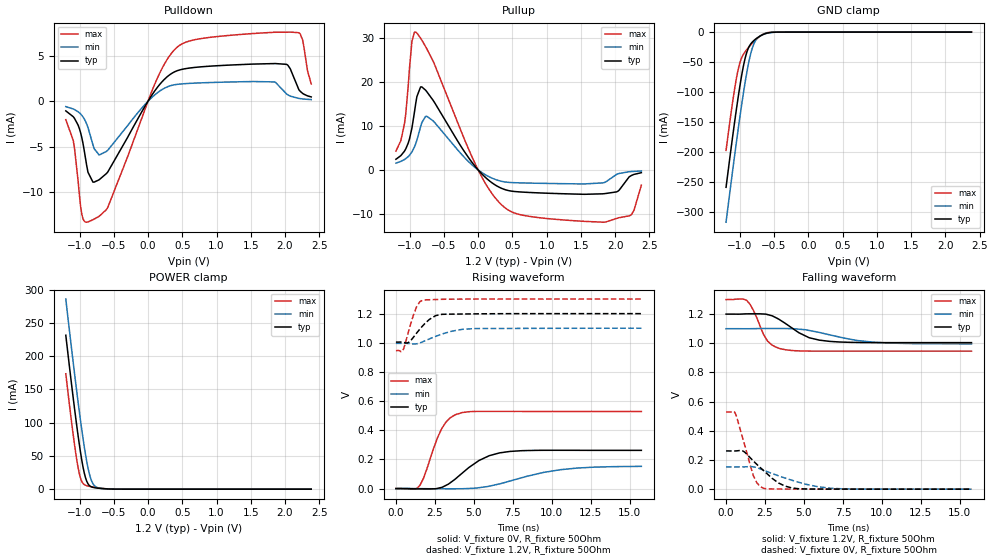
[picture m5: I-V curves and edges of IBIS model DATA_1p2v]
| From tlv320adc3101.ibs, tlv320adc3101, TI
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|   DATA_1p2v
[Model]   DATA_1p2v
Model_type   3-state
Polarity   Non-Inverting
Vmeas = 0.6
Vref = 0
Cref = 5pF
Rref = 1000000
|   typ   min   max
C_comp   1.339pF   1.297pF   1.403pF
[Voltage Range]   1.2   1.1   1.3
[Temperature Range]   27   85   -40
[Pullup Reference]   1.2   1.1   1.3
[Pulldown Reference]   -0   -0   -0
[Power Clamp Reference]   1.2   1.1   1.3
[GND Clamp Reference]   -0   -0   -0
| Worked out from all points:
|   slope of the pulldown table from 0 to 0.18 V, typ, clamps not added: 93.3 ohm
|   slope of the pullup table from 0 to 0.18 V, typ, clamps not added: 67.6 ohm
|   GND clamp passes 1 mA (typ) near -0.57 V on its own axis
|   POWER clamp passes 1 mA (typ) near -0.68 V on its own axis
|   falling waveform, V_fixture 1.2V, R_fixture 50Ohm: 20-80 % time 1.78ns typ, 2.86ns min, 916ps max; typ from 1.2 V to 1 V
|   rising waveform, V_fixture 0V, R_fixture 50Ohm: 20-80 % time 2.02ns typ, 3.54ns min, 1.12ns max; typ from 0 V to 0.262 V
|   rising waveform, V_fixture 1.2V, R_fixture 50Ohm: 20-80 % time 992ps typ, 1.64ns min, 608ps max; typ from 1 V to 1.2 V
|   falling waveform, V_fixture 0V, R_fixture 50Ohm: 20-80 % time 1.63ns typ, 2.66ns min, 845ps max; typ from 0.262 V to 0 V
[Pulldown]
|   Voltage   I(typ)   I(min)   I(max)
-1.2V     -1.067mA   -596.5uA   -2.034mA
-1.092V   -1.704mA   -854.7uA   -4.302mA
-1.02V    -2.641mA   -1.168mA   -8.814mA
-966mV    -4.025mA   -1.562mA   -12.47mA
-894mV    -7.132mA   -2.535mA   -13.33mA
-714mV    -8.661mA   -5.927mA   -12.69mA
-588mV    -7.809mA   -5.412mA   -11.72mA
168mV     1.822mA    1.102mA    3.055mA
492mV     3.504mA    1.906mA    6.299mA
2.022V    4.063mA    801.9uA    7.609mA
2.202V    1.263mA    305.2uA    7.544mA
2.382V    470uA      178.4uA    1.899mA
[GND Clamp]
|   Voltage   I(typ)   I(min)   I(max)
-1.2V     -258.3mA   -316.3mA   -196.8mA
-1.11V    -179.2mA   -235.9mA   -121mA
-1.038V   -119.9mA   -174.1mA   -70.4mA
-984mV    -80.01mA   -130.2mA   -46.12mA
-930mV    -47.6mA    -89.49mA   -34.07mA
-876mV    -27.11mA   -54.39mA   -26.08mA
-822mV    -17.22mA   -28.43mA   -19.08mA
-768mV    -11.59mA   -13.93mA   -12.83mA
-714mV    -7.351mA   -7.4mA     -7.548mA
-624mV    -2.47mA    -2.583mA   -1.855mA
-534mV    -437.8uA   -605.1uA   -188uA
2.382V    0A         0A         0A
[Pullup]
|   Voltage   I(typ)   I(min)   I(max)
-1.2V     2.416mA    1.543mA    4.264mA
-1.074V   4.282mA    2.371mA    10.56mA
-966mV    9.533mA    4.093mA    29.21mA
-912mV    14.96mA    5.898mA    31.25mA
-840mV    18.81mA    9.781mA    29.89mA
-750mV    17.75mA    12.16mA    27.48mA
6mV       -105.3uA   -68.85uA   -187.8uA
420mV     -4.595mA   -2.784mA   -8.894mA
1.86V     -5.351mA   -2.743mA   -11.81mA
2.04V     -4.824mA   -892.5uA   -10.9mA
2.238V    -1.257mA   -368.2uA   -10.12mA
2.382V    -625.5uA   -250uA     -3.472mA
[POWER Clamp]
|   Voltage   I(typ)   I(min)   I(max)
-1.2V     231.5mA    285.9mA    173.6mA
-1.128V   168mA      221.8mA    111.1mA
-1.074V   122.5mA    175.2mA    67.98mA
-1.038V   93.72mA    145.2mA    42.82mA
-1.002V   66.93mA    116.2mA    23.06mA
-948mV    32.97mA    75.79mA    8.518mA
-894mV    11.73mA    41.39mA    5.177mA
-840mV    4.19mA     17.16mA    3.878mA
-804mV    2.69mA     8.241mA    3.201mA
-768mV    1.973mA    3.956mA    2.587mA
-480mV    51.54uA    83.66uA    36.66uA
2.382V    0A         0A         0A
[Ramp]
R_load = 50
|   typ   min   max
dV/dt_r   0.157258/2.02351e-009 0.0913677/3.53646e-009  0.317481/1.12489e-009
dV/dt_f   0.117245/1.77819e-009  0.062355/2.86362e-009  0.212218/9.16152e-010
[Falling Waveform]
V_fixture = 1.2V
V_fixture_min = 1.1V
V_fixture_max = 1.3V
R_fixture = 50Ohm
C_fixture = 0F
|   Time   V(typ)   V(min)   V(max)
0s        1.2V       1.1V       1.3V
1.323ns   1.202V     1.1V       1.295V
1.757ns   1.202V     1.1V       1.226V
2.407ns   1.201V     1.101V     1.06V
2.671ns   1.197V     1.101V     1.014V
3.8ns     1.137V     1.101V     955.9mV
5.33ns    1.038V     1.088V     946.6mV
6.649ns   1.013V     1.058V     946.2mV
9.482ns   1.005V     1.007V     946.3mV
15.74ns   1.005V     996.1mV    946.3mV
[Rising Waveform]
V_fixture = 0V
V_fixture_min = 0V
V_fixture_max = 0V
R_fixture = 50Ohm
C_fixture = 0F
|   Time   V(typ)   V(min)   V(max)
0s        -5.034uV   -4.456uV   -11.14uV
1.107ns   -1.549mV   133uV      -4.132mV
1.54ns    -2.225mV   -325.2uV   21.68mV
2.935ns   7.885mV    -1.35mV    410.4mV
3.463ns   37.93mV    -1.431mV   483.6mV
3.8ns     64.69mV    -1.379mV   506.3mV
5.33ns    192.6mV    6.037mV    529.4mV
6.649ns   244.8mV    32.23mV    529.4mV
10.56ns   262.6mV    129.5mV    529.1mV
15.74ns   262.1mV    152.3mV    529.1mV
[Rising Waveform]
V_fixture = 1.2V
V_fixture_min = 1.1V
V_fixture_max = 1.3V
R_fixture = 50Ohm
C_fixture = 0F
|   Time   V(typ)   V(min)   V(max)
0s        1.005V     996.1mV    946.4mV
433.2ps   1.004V     996.5mV    945.1mV
842ps     1.005V     995mV      1.09V
1.323ns   1.066V     993.2mV    1.246V
1.54ns    1.095V     999.5mV    1.283V
1.757ns   1.121V     1.009V     1.293V
2.553ns   1.187V     1.044V     1.297V
2.96ns    1.195V     1.06V      1.298V
5.079ns   1.198V     1.098V     1.3V
15.74ns   1.2V       1.1V       1.3V
[Falling Waveform]
|Gnd
V_fixture = 0V
V_fixture_min = 0V
V_fixture_max = 0V
R_fixture = 50Ohm
C_fixture = 0F
|   Time   V(typ)   V(min)   V(max)
0s        262.1mV    152.5mV    529.1mV
582.4ps   262mV      152.3mV    522.4mV
1.069ns   262.3mV    152.6mV    349.3mV
1.757ns   192.8mV    153mV      91.59mV
1.973ns   170.2mV    147.6mV    44.3mV
2.407ns   127.5mV    130.3mV    5.662mV
3.367ns   42.39mV    91.44mV    1.139mV
4.67ns    2.675mV    47.15mV    124.3uV
7.571ns   296.2uV    1.857mV    2.695uV
15.74ns   -1.281uV   17.98uV    118.9nV
